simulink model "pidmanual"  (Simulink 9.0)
settings: Solver=VariableStepAuto  StartTime=0.0  StopTime=dps_simdata.endTime  RelTol=1e-3
undefined symbols (not defined in the file or in its folder): dps_simdata
libraries: dps x5

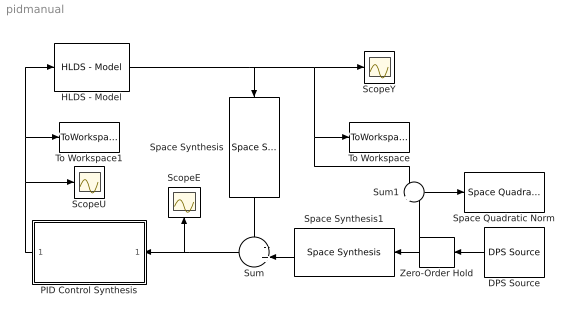
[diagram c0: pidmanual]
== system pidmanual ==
  DPS Source : dps/DPS Source  equation=dps_simdata.w  responseVar=0  showInput=off  pointsCoord=dps_simdata.points  elementsVar=[]  samplePeriod=dps_simdata.T
  HLDS - Model : dps/Controlled Systems/HLDS - Model  StepResponse=dps_simdata.H  samplePeriod=dps_simdata.T  u_step=1
  PID Control Synthesis : Subsystem  AncestorBlock=dps/Temporal Synthesis/PID Control Synthesis
  ScopeE : Scope
  ScopeU : Scope
  ScopeY : Scope
  Space Quadratic Norm : dps/Quadratic norms/Space Quadratic Norm  StepResponse=dps_simdata.H  showNorm=on
  Space Synthesis : dps/Space Synthesis/Space Synthesis  PCH=dps_simdata.H  weights=dps_simdata.weights
  Space Synthesis1 : dps/Space Synthesis/Space Synthesis  PCH=dps_simdata.H  weights=dps_simdata.weights
  Sum : Sum  Inputs=-+|
  Sum1 : Sum  Inputs=-|+
  To Workspace : ToWorkspace  VariableName=simY  SaveFormat=Structure  SampleTime=-1
  To Workspace1 : ToWorkspace  VariableName=simU  SaveFormat=Structure  SampleTime=-1
  Zero-Order Hold : ZeroOrderHold  SampleTime=-1
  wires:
  HLDS - Model/1 -> Sum1/1, To Workspace/1, ScopeY/1, Space Synthesis/1
  PID Control Synthesis/1(u) -> HLDS - Model/1, To Workspace1/1, ScopeU/1
  DPS Source/1 -> Zero-Order Hold/1
  Sum/1 -> PID Control Synthesis/1(e), ScopeE/1
  Zero-Order Hold/1 -> Sum1/2, Space Synthesis1/1
  Space Synthesis/1 -> Sum/1
  Space Synthesis1/1 -> Sum/2
  Sum1/1 -> Space Quadratic Norm/1

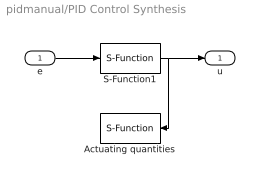
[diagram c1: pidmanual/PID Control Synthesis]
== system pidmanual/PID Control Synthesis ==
  e : Inport
  Actuating quantities : S-Function  FunctionName=sfun_scope  Parameters=length(dps_simdata.H)  SFunctionDeploymentMode=off  EnableBusSupport=off
  S-Function1 : S-Function  FunctionName=sfun_psd  Parameters='method',method,'num',b,'den',a,'P',r0,'I',ri,'D',rd,'TAU',tau,'samplePeriod',samplePeriod,'weights',weights,'StepResponse',StepResponse  SFunctionDeploymentMode=off  EnableBusSupport=off
  u : Outport
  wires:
  e/1 -> S-Function1/1
  S-Function1/1 -> u/1, Actuating quantities/1
